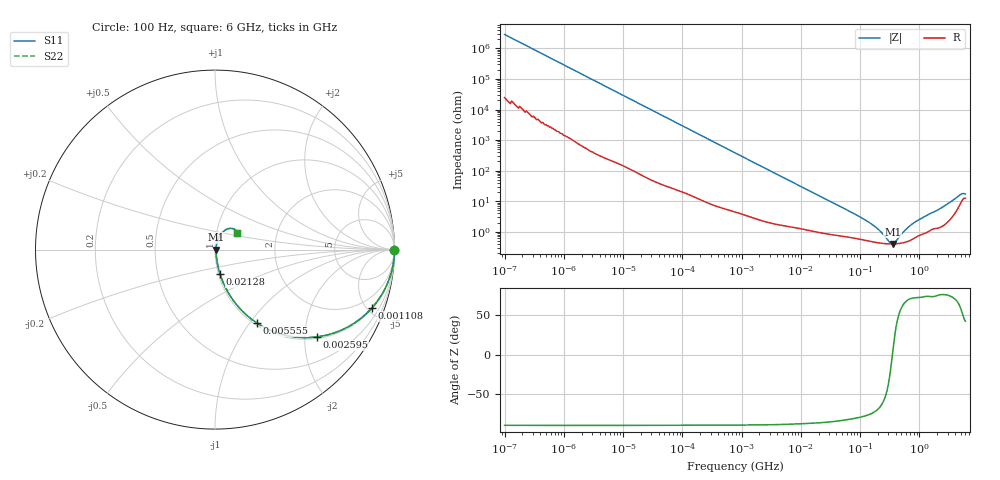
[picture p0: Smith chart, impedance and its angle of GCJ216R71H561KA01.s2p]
!Murata Part Number: GCJ216R71H561KA01
!These Parameters are Measured in Series Mode Connection
!Data Generated on Mar 13, 2026
!  o--ll--o
!Port1  Port2
!  o------o
!Operation Temp=25[degC], DC Bias Voltage=0[V]
!Freq. Start=100[Hz] Stop=6[GHz] 401[Steps]
# Hz S RI R 50
!Freq.(Hz) S11(Real) S11(Imag) S21(Real) S21(Imag) S12(Real) S12(Imag) S22(Real) S22(Imag)
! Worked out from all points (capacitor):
!   401 points, 100 Hz to 6 GHz, reference 50 ohm
!   read as one part in series: C = 556 pF near 109 Hz
!   lowest |Z| = 400 mohm at 357.3 MHz (marker M1)
!   series resonance near 351.3 MHz, so ESL is about 370 pH
!   S11 on the Smith chart (normalised r, x): 100 Hz: open; 1.108 MHz: 1.07, -5.34; 2.595 MHz: 1.04, -2.29; 5.555 MHz: 1.03, -1.08; 21.28 MHz: 1.02, -0.29; 6 GHz: 1.25, +0.23
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100  1 -3.5e-05  3e-07 3.5e-05  3e-07 3.5e-05  1 -3.5e-05
293  1 -0.000102  6e-07 0.000102  6e-07 0.000102  1 -0.000102
2008  1 -0.000695  3.6e-06 0.000695  3.6e-06 0.000695  1 -0.000695
40335  0.9997 -0.0138  0.000264 0.0138  0.000264 0.0138  0.9997 -0.0138
231233  0.9932 -0.0782  0.00677 0.0782  0.00677 0.0782  0.9932 -0.0782
774597  0.933 -0.2442  0.067 0.2442  0.067 0.2442  0.933 -0.2442
1108252  0.8736 -0.3257  0.1264 0.3257  0.1264 0.3257  0.8736 -0.3257
2594782  0.5668 -0.4865  0.4332 0.4865  0.4332 0.4865  0.5668 -0.4865
5554849  0.2314 -0.4077  0.7686 0.4077  0.7686 0.4077  0.2314 -0.4077
8692127  0.1162 -0.302  0.8838 0.302  0.8838 0.302  0.1162 -0.302
1.555665e7  0.046 -0.1844  0.954 0.1844  0.954 0.1844  0.046 -0.1844
2.128304e7  0.0288 -0.138  0.9712 0.138  0.9712 0.138  0.0288 -0.138
1.395531e8  0.00531 -0.0199  0.9947 0.0199  0.9947 0.0199  0.00531 -0.0199
2.088084e8  0.00438 -0.0104  0.9956 0.0104  0.9956 0.0104  0.00438 -0.0104
3.124326e8  0.00398 -0.00229  0.996 0.00229  0.996 0.00229  0.00398 -0.00229
3.573489e8  0.00397 0.000338  0.996 -0.000338  0.996 -0.000338  0.00397 0.000338
3.908258e8  0.004 0.0021  0.996 -0.0021  0.996 -0.0021  0.004 0.0021
6.11557e8  0.00478 0.0116  0.9952 -0.0116  0.9952 -0.0116  0.00478 0.0116
8.366708e8  0.00658 0.0192  0.9934 -0.0192  0.9934 -0.0192  0.00658 0.0192
2.931063e9  0.0247 0.0731  0.9753 -0.0731  0.9753 -0.0731  0.0247 0.0731
4.796499e9  0.0839 0.1183  0.9161 -0.1183  0.9161 -0.1183  0.0839 0.1183
6e9  0.1212 0.0904  0.8788 -0.0904  0.8788 -0.0904  0.1212 0.0904
